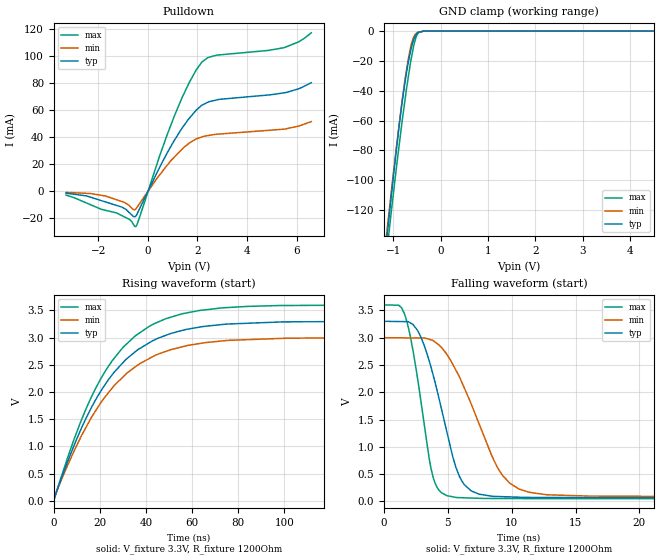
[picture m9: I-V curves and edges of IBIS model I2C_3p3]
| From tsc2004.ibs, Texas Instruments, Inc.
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| Model 3.3 V I2C
[Model]   I2C_3p3
Model_type   I/O_open_drain
Polarity   Non-Inverting
Enable   Active-Low
Vinl = 0.99
Vinh = 2.31
Vmeas = 1.65
Vref = 1.65
Cref = 15pF
Rref = 1200
|   typ   min   max
|   (nom PVT)   (Fast PVT)   (slow PVT)
|   Output High
C_comp   1.2305E-11   1.2305E-11   1.2305E-11
|   Output Low
|C_comp   1.20804E-11   1.16972E-11   1.2305E-11
| Where   nom PVT is  Nominal Process, 3.3V, 25C
|   Fast PVT is Strong Process, 3.6V, -40C
|   Slow PVT is Weak Process, 3.0V, 85C
|C_comp - from L-C Tank method, L = 1nH, peak frequency ~ 1.45GHz
[Model Spec]   | power 3.3. 3, 3.6 V
Vinl   0.99   0.9   1.08
Vinh   2.31   2.1   2.52
[Voltage Range]   3.3   3   3.6
[Temperature Range]   30   88   -40
|Ambient Temperature Range 27   85   -40
[Pullup Reference]   3.3   3   3.6
[Pulldown Reference]   0   0   0
[Power Clamp Reference]   3.3   3   3.6
[GND Clamp Reference]   0   0   0
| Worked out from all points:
|   slope of the pulldown table from 0 to 0.495 V, typ, clamps not added: 26.5 ohm
|   GND clamp passes 1 mA (typ) near -0.48 V on its own axis
|   falling waveform, V_fixture 3.3V, R_fixture 1200Ohm: 20-80 % time 2.08ns typ, 3.18ns min, 1.39ns max; typ from 3.3 V to 0.069 V
|   rising waveform, V_fixture 3.3V, R_fixture 1200Ohm: 20-80 % time 26.9ns typ, 27.8ns min, 26.1ns max; typ from 0.069 V to 3.3 V
[Pulldown]
|   Voltage   I(typ)   I(min)   I(max)
-3.3V     -1.293mA   -705.8uA   -2.704mA
-1.711V   -7.756mA   -3.38mA    -13.98mA
-1.061V   -11.52mA   -7.372mA   -17.79mA
-740.5mV  -15.86mA   -10.69mA   -20.75mA
-490mV    -18.25mA   -13.03mA   -26.03mA
475.5mV   17.99mA    12.3mA     26.46mA
1.076V    38.11mA    25.62mA    56.3mA
1.676V    54.36mA    35.9mA     80.99mA
2.178V    63.84mA    40.38mA    95.86mA
2.767V    67.75mA    42.36mA    100.9mA
5.498V    73.07mA    46.16mA    106.5mA
6.59V     80.55mA    51.7mA     117.5mA
[GND Clamp]
|   Voltage   I(typ)   I(min)   I(max)
-3.3V     -849.8mA   -809.8mA   -887mA
-1.157V   -144.1mA   -139.5mA   -153.3mA
-1.128V   -135.2mA   -131mA     -144.8mA
-1.072V   -118.1mA   -115mA     -128.4mA
-894.1mV  -67.31mA   -66.21mA   -80.14mA
-755.7mV  -34.11mA   -32.48mA   -45.97mA
-685mV    -20.58mA   -18.31mA   -30.46mA
-613.4mV  -10.08mA   -7.745mA   -16.61mA
-549.7mV  -3.927mA   -2.696mA   -6.94mA
-495.3mV  -1.398mA   -851.7uA   -2.273mA
-350mV    -26.57uA   -25.44uA   -16.78uA
6.59V     0A         0A         0A
[POWER Clamp]
|   SCR cell for ESD function. Effects occurr above VDD x 2
|   Voltage   I(typ)   I(min)   I(max)
-3.3V     0A         0A         0A
0V        0A         0A         0A
6.6V      0A         0A         0A
[Ramp]
R_load = 1200
|   typ   min   max
dV/dt_r   1.93851/2.68225e-008   1.74633/2.76231e-008   2.12897/2.59184e-008
dV/dt_f   1.93851/2.0706e-009   1.74633/3.15462e-009   2.12898/1.38365e-009
[Falling Waveform]
V_fixture = 3.3V
V_fixture_min = 3V
V_fixture_max = 3.6V
R_fixture = 1200Ohm
C_fixture = 0F
|   Time   V(typ)   V(min)   V(max)
0s        3.299V     2.999V     3.6V
1.587ns   3.294V     2.996V     3.445V
2.738ns   3.084V     2.994V     2.083V
3.517ns   2.59V      2.972V     816.8mV
3.978ns   2.199V     2.922V     348.5mV
5.656ns   610mV      2.392V     73.94mV
6.806ns   198.5mV    1.799V     63.44mV
9.256ns   88.74mV    484.7mV    54.83mV
12.83ns   73.59mV    122.6mV    51.77mV
150ns     68.61mV    88.81mV    51.29mV
[Rising Waveform]
V_fixture = 3.3V
V_fixture_min = 3V
V_fixture_max = 3.6V
R_fixture = 1200Ohm
C_fixture = 0F
|   Time   V(typ)   V(min)   V(max)
0s        68.61mV    88.81mV    51.29mV
467.6ps   76.67mV    84.89mV    69.86mV
5.805ns   699.8mV    634.4mV    771.1mV
11.49ns   1.287V     1.153V     1.434V
20.19ns   2.001V     1.789V     2.229V
29.96ns   2.538V     2.274V     2.816V
41.4ns    2.903V     2.614V     3.205V
55.39ns   3.127V     2.827V     3.433V
72.5ns    3.237V     2.935V     3.543V
150ns     3.299V     2.999V     3.6V
